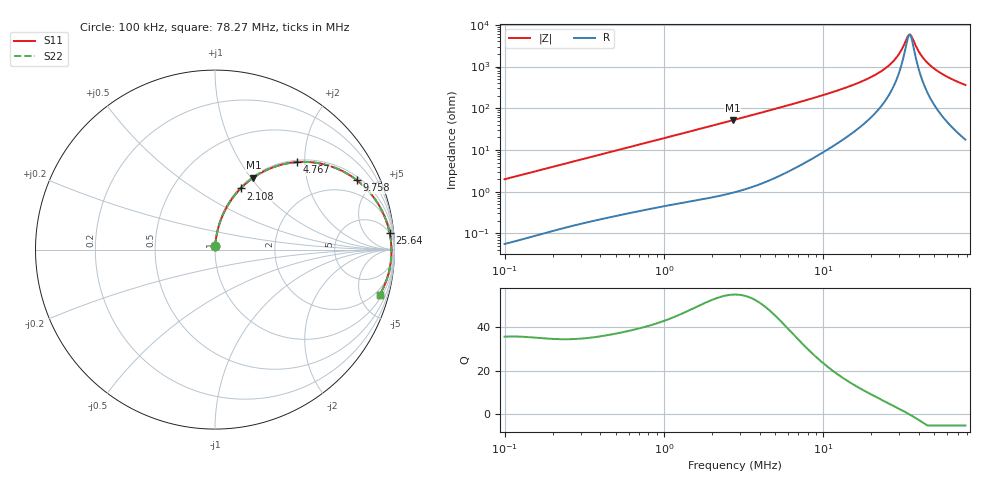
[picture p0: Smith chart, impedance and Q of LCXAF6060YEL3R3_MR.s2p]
! LCXAF6060YEL3R3_MR  S-PARAMETER MODEL  ( General Type )
! Model Generated by TAIYO YUDEN Corporation (http://www.ty-top.com)
! Version 1.0
! TAIYO YUDEN Control No. 200406NI43SB-FBB
! Copyright(c) 2020 TAIYO YUDEN CO.,LTD. All Rights Reserved.
! Product Description (link to TY-COMPAS)
! https://ds.yuden.co.jp/TYCOMPAS/or/detail?pn=LCXAF6060YEL3R3MMR&u=M
! Products Name : Inductors
! Characteristics :
!  Inductance : 3.3 uH , SRF(min) : 24 MHz , DC Resistance(max) : 0.032 Ohm
!  Rated Current : Saturation :9000 mA , Temp Rise : 3800 mA (40 degC)
!  Case Size : 6.0 x 6.0 / 0.236 x 0.236 [mm/inch] , Thickness : 4.5 / 0.177 [mm/inch]
!  (Conditions: Temperature = 25 degC , DC Bias Current/Voltage = 0A / 0V)
! External Node Assignments :
!  1  o---GGG---o  2
! GND o---------o GND
! Frequency Range : 0.1MHz  -  78.268192MHz  [ 402 STEP ]
# MHz S RI R 50
! Freq[MHz].  S11 Real  S11 Imag  S21 Real  S21 Imag  S12 Real  S12 Imag  S22 Real  S22 Imag
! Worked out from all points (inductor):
!   401 points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, 100 kHz to 78.27 MHz, reference 50 ohm
!   read as one part in series: L = 3.15 uH near 103.4 kHz
!   highest Q = 54.7 at 2.706 MHz (marker M1), where L = 3.03 uH
!   self-resonance near 34.6 MHz
!   S11 on the Smith chart (normalised r, x): 100 kHz: 1.00, +0.04; 2.108 MHz: 1.02, +0.80; 4.767 MHz: 1.04, +1.84; 9.758 MHz: 1.17, +4.00; 25.64 MHz: 5, +20; 78.27 MHz: 1.35, -7.20
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0.1  0.000953 0.0198  0.999 -0.0198  0.999 -0.0198  0.000953 0.0198
0.305264  0.00523 0.0591  0.9948 -0.0591  0.9948 -0.0591  0.00523 0.0591
0.931861  0.0346 0.1713  0.9654 -0.1713  0.9654 -0.1713  0.0346 0.1713
2.107731  0.143 0.3407  0.857 -0.3407  0.857 -0.3407  0.143 0.3407
2.705981  0.2139 0.401  0.7861 -0.401  0.7861 -0.401  0.2139 0.401
2.844635  0.231 0.4124  0.769 -0.4124  0.769 -0.4124  0.231 0.4124
4.767377  0.4588 0.4877  0.5412 -0.4877  0.5412 -0.4877  0.4588 0.4877
8.540203  0.7398 0.4212  0.2602 -0.4212  0.2602 -0.4212  0.7398 0.4212
9.75753  0.7908 0.3865  0.2092 -0.3865  0.2092 -0.3865  0.7908 0.3865
17.77307  0.9367 0.2029  0.0633 -0.2029  0.0633 -0.2029  0.9367 0.2029
21.70552  0.9604 0.1415  0.0396 -0.1415  0.0396 -0.1415  0.9604 0.1415
25.63951  0.9733 0.0915  0.0267 -0.0915  0.0267 -0.0915  0.9733 0.0915
26.07016  0.9743 0.0866  0.0257 -0.0866  0.0257 -0.0866  0.9743 0.0866
29.29419  0.9797 0.0521  0.0203 -0.0521  0.0203 -0.0521  0.9797 0.0521
31.31247  0.9817 0.0324  0.0183 -0.0324  0.0183 -0.0324  0.9817 0.0324
34.03197  0.9831 0.00786  0.0169 -0.00786  0.0169 -0.00786  0.9831 0.00786
35.1848  0.9833 -0.00199  0.0167 0.00199  0.0167 0.00199  0.9833 -0.00199
36.37667  0.9834 -0.0119  0.0166 0.0119  0.0166 0.0119  0.9834 -0.0119
41.56183  0.9814 -0.0516  0.0186 0.0516  0.0186 0.0516  0.9814 -0.0516
47.48609  0.9761 -0.092  0.0239 0.092  0.0239 0.092  0.9761 -0.092
58.96685  0.9591 -0.1595  0.0409 0.1595  0.0409 0.1595  0.9591 -0.1595
78.26819  0.9179 -0.2511  0.0821 0.2511  0.0821 0.2511  0.9179 -0.2511
